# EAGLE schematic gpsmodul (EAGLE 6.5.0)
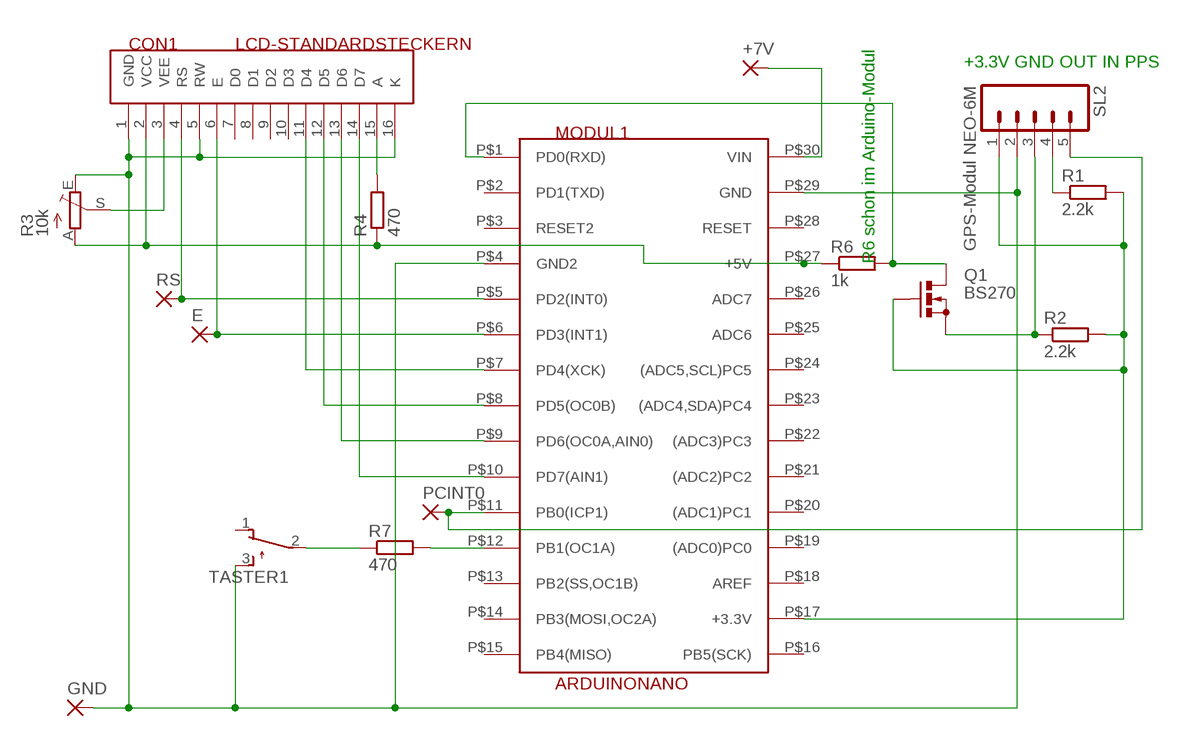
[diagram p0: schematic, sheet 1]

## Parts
+7V  1,6/0,8  [1,6/0,8]
CON1  LCD-STANDARDSTECKERN  [STECKER16]
E  1,6/0,8  [1,6/0,8]
GND  1,6/0,8  [1,6/0,8]
MODUL1  ARDUINONANO  [ARDUINONANO]
PCINT0  1,6/0,8  [1,6/0,8]
Q1  BS270  BS170  [SOT54E]
R1  2.2k  R-EU_0204/7  [0204/7]
R2  2.2k  R-EU_0204/7  [0204/7]
R3  10k  TRIM_EU-B64W  [B64W]
R4  470  R-EU_0204/7  [0204/7]
R6  1k  R-EU_0204/7  [0204/7]
R7  470  R-EU_0204/7  [0204/7]
RS  1,6/0,8  [1,6/0,8]
SL2  GPS-Modul NEO-6M  M05  [05P]
TASTER1  TL32PO  [TL3XPO]

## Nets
GND: CON1.1(GND) CON1.5(RW) CON1.16(K) GND.1(P) MODUL1.P$4(GND2) MODUL1.P$29(GND) R3.E SL2.2 TASTER1.3(S)
N$1: MODUL1.P$1(PD0(RXD)) Q1.D R6.2
N$2: Q1.S R2.1 SL2.3
N$4: R1.1 SL2.4
N$5: MODUL1.P$11(PB0(ICP1)) PCINT0.1(P) SL2.5
N$6: CON1.15(A) R4.2
N$7: CON1.3(VEE) R3.S
N$8: CON1.14(D7) MODUL1.P$10(PD7(AIN1))
N$9: CON1.13(D6) MODUL1.P$9(PD6(OC0A,AIN0))
N$10: CON1.12(D5) MODUL1.P$8(PD5(OC0B))
N$11: CON1.11(D4) MODUL1.P$7(PD4(XCK))
N$12: CON1.6(E) E.1(P) MODUL1.P$6(PD3(INT1))
N$13: CON1.4(RS) MODUL1.P$5(PD2(INT0)) RS.1(P)
N$14: R7.1 TASTER1.2(P)
N$15: MODUL1.P$12(PB1(OC1A)) R7.2
V3.3: MODUL1.P$17(+3.3V) Q1.G R1.2 R2.2 SL2.1
VCC: CON1.2(VCC) MODUL1.P$27(+5V) R3.A R4.1 R6.1
VIN: +7V.1(P) MODUL1.P$30(VIN)
Unconnected: CON1.7(D0) CON1.8(D1) CON1.9(D2) CON1.10(D3) MODUL1.P$2(PD1(TXD)) MODUL1.P$3(RESET2) MODUL1.P$13(PB2(SS,OC1B)) MODUL1.P$14(PB3(MOSI,OC2A)) MODUL1.P$15(PB4(MISO)) MODUL1.P$16(PB5(SCK)) MODUL1.P$18(AREF) MODUL1.P$19((ADC0)PC0) MODUL1.P$20((ADC1)PC1) MODUL1.P$21((ADC2)PC2) MODUL1.P$22((ADC3)PC3) MODUL1.P$23((ADC4,SDA)PC4) MODUL1.P$24((ADC5,SCL)PC5) MODUL1.P$25(ADC6) MODUL1.P$26(ADC7) MODUL1.P$28(RESET) TASTER1.1(O)

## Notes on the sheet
- +3.3V GND OUT IN PPS
- R6 schon im Arduino-Modul

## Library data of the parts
+7V E GND PCINT0 RS = wirepad:1,6/0,8: THROUGH-HOLE PAD
CON1 = 6_stecker:LCD-STANDARDSTECKER: Standard-Stecker fuer die meisten LCD-Module
MODUL1 = arduino:ARDUINONANO
Q1 = transistor-small-signal:BS170: N-CHANNEL MOS FET
R1 R2 R4 R6 R7 = rcl:R-EU_: RESISTOR, European symbol
R3 = pot:TRIM_EU-: POTENTIOMETER
SL2 = con-amp-quick:M05: AMP QUICK CONNECTOR; OC_FARNELL: unknown; OC_NEWARK: unknown
TASTER1 = switch:TL32PO: TINY SWITCH ON - MOM Source: http://www2.produktinfo.conrad.com/datenblaetter/700000-724999/705152-da-01-de-Subminiaturschalter_TL_36YO.pdf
